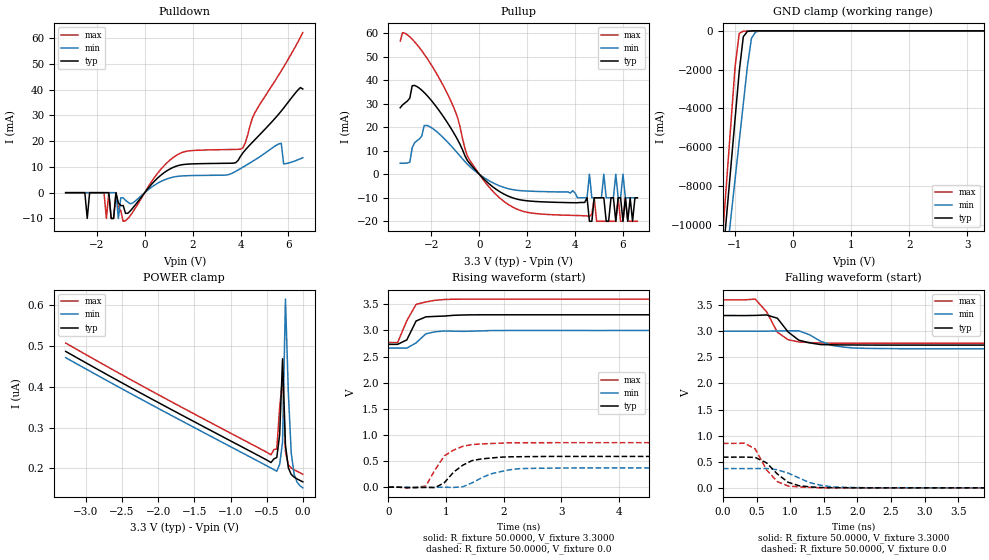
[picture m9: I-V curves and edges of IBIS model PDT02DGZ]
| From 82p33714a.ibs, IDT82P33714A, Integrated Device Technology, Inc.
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|   Model PDT02DGZ@
[Model]  PDT02DGZ
Model_type 3-state
Polarity   Non-Inverting
Enable   Active-Low
Vmeas =  1.6500V
Cref =   50.0000pF
Rref =   1.0000M
Vref =   0.0V
C_comp   70.4000fF   58.1000fF   75.7000fF
[Temperature Range]   25.0000   0.1250k   -40.0000
[Voltage Range]   3.3000V   3.0000V   3.6000V
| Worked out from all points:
|   slope of the pulldown table from 0 to 0.495 V, typ, clamps not added: 93.5 ohm
|   slope of the pullup table from 0 to 0.495 V, typ, clamps not added: 103 ohm
|   GND clamp passes 1 mA (typ) near -0.64 V on its own axis
|   rising waveform, R_fixture 50.0000, V_fixture 3.3000: 20-80 % time 160ps typ, 217ps min, 223ps max; typ from 2.73 V to 3.3 V
|   rising waveform, R_fixture 50.0000, V_fixture 0.0: 20-80 % time 384ps typ, 503ps min, 363ps max; typ from 0 V to 0.588 V
|   falling waveform, R_fixture 50.0000, V_fixture 3.3000: 20-80 % time 262ps typ, 328ps min, 254ps max; typ from 3.3 V to 2.73 V
|   falling waveform, R_fixture 50.0000, V_fixture 0.0: 20-80 % time 304ps typ, 438ps min, 266ps max; typ from 0.588 V to 0 V
[Pulldown]
|Voltage   I(typ)   I(min)   I(max)
-3.3V     0A         0A         0A
-2.5V     0A         0A         0A
-2.4V     -10mA      0A         0A
-1.6V     0A         0A         -10mA
-1.5V     0A         0A         0A
-1.4V     -10mA      0A         -10mA
-1.2V     0A         0A         0A
-1.1V     -4mA       -10mA      -6mA
-900mV    -5mA       -2mA       -11.11mA
1.3V      10.23mA    6.236mA    14.35mA
4.1V      15.46mA    9.888mA    17.41mA
6.6V      40.22mA    13.56mA    62.13mA
[Pullup]
|Voltage   I(typ)   I(min)   I(max)
-3.3V     28.25mA    4.655mA    56.59mA
-2.2V     33.66mA    20.75mA    49.56mA
-400mV    4.59mA     3.281mA    5.938mA
1V        -8.271mA   -5.504mA   -11.3mA
4.5V      -10mA      -10mA      -17.7mA
4.6V      -20mA      0A         -18mA
4.7V      -20mA      -10mA      -17mA
4.8V      -10mA      -10mA      -10mA
6V        -20mA      0A         -20mA
6.1V      -10mA      -10mA      -10mA
6.2V      -20mA      -10mA      -20mA
6.6V      -10mA      -10mA      -20mA
[GND_clamp]
|Voltage   I(typ)   I(min)   I(max)
-3.3V     -83.46A    -71.04A    -95.7A
-1.2V     -11.69A    -13.39A    -10.37A
-1.13V    -9.3A      -11.47A    -7.522A
-1.06V    -6.904A    -9.549A    -4.675A
-990mV    -4.509A    -7.624A    -1.828A
-920mV    -2.113A    -5.699A    -140.7mA
-850mV    -308.3mA   -3.775A    -17.61mA
-780mV    -30.18mA   -1.85A     -8.684mA
-710mV    -4.231mA   -388.3mA   -4.536mA
-640mV    -826.8uA   -62.95mA   -1.713mA
-430mV    -4.377uA   -246.1uA   -5.398uA
3.28V     165.3nA    264.6nA    156.9nA
[POWER_clamp]
|Voltage   I(typ)   I(min)   I(max)
-3.28V    486.2nA    470.9nA    506.6nA
-440mV    214.3nA    200.8nA    233.1nA
-400mV    223.3nA    196.9nA    246nA
-360mV    226.7nA    193nA      247.8nA
-320mV    282.8nA    210nA      349.4nA
-280mV    468.1nA    264.6nA    421.2nA
-240mV    257.3nA    614.1nA    241nA
-200mV    201.3nA    384.8nA    208.8nA
-160mV    185.2nA    237.6nA    200.8nA
-120mV    178.7nA    185.9nA    196.6nA
-80mV     174.4nA    166.5nA    192.9nA
0V        167.1nA    152.4nA    185.7nA
[Ramp]
| variable   typ   min   max
dV/dt_r  0.3530/0.3844n   0.2212/0.4930n   0.5110/0.3630n
dV/dt_f  0.3396/0.2623n   0.2022/0.3186n   0.4986/0.2510n
R_load = 50.0000
[Rising Waveform]
R_fixture= 50.0000
V_fixture= 3.3000
V_fixture_min= 3.0000
V_fixture_max= 3.6000
L_fixture= 0.0H
C_fixture= 0.0F
|time   V(typ)   V(min)   V(max)
0s        2.734V     2.663V     2.769V
160ps     2.734V     2.663V     2.768V
320ps     2.82V      2.662V     3.188V
480ps     3.181V     2.762V     3.499V
650ps     3.261V     2.936V     3.546V
810ps     3.269V     2.975V     3.578V
970ps     3.276V     2.99V      3.593V
1.29ns    3.296V     2.983V     3.599V
1.62ns    3.3V       2.992V     3.599V
16ns      3.3V       3V         3.6V
[Rising Waveform]
R_fixture= 50.0000
V_fixture= 0.0
V_fixture_min= 0.0
V_fixture_max= 0.0
L_fixture= 0.0H
C_fixture= 0.0F
|time   V(typ)   V(min)   V(max)
0s        7.011uV    7.347uV    6.889uV
650ps     -2.872mV   -5.444mV   22.73mV
810ps     -8.827mV   -2.518mV   335.1mV
970ps     85.14mV    -1.489mV   599.3mV
1.13ns    288.1mV    -5.225mV   709.9mV
1.29ns    421.3mV    8.1mV      782.5mV
1.62ns    541.9mV    182.4mV    828.5mV
2.1ns     581mV      332.4mV    850.5mV
2.59ns    586.5mV    361.9mV    851.3mV
16ns      588.4mV    368.7mV    851.6mV
[Falling Waveform]
R_fixture= 50.0000
V_fixture= 3.3000
V_fixture_min= 3.0000
V_fixture_max= 3.6000
L_fixture= 0.0H
C_fixture= 0.0F
|time   V(typ)   V(min)   V(max)
0s        3.3V       3V         3.6V
480ps     3.302V     2.999V     3.614V
650ps     3.311V     3V         3.372V
810ps     3.248V     3.004V     2.98V
970ps     2.985V     3.007V     2.837V
1.13ns    2.827V     3.007V     2.794V
1.45ns    2.744V     2.809V     2.773V
1.78ns    2.737V     2.698V     2.77V
2.59ns    2.734V     2.665V     2.769V
16ns      2.734V     2.663V     2.769V
[Falling Waveform]
R_fixture= 50.0000
V_fixture= 0.0
V_fixture_min= 0.0
V_fixture_max= 0.0
L_fixture= 0.0H
C_fixture= 0.0F
|time   V(typ)   V(min)   V(max)
0s        588.4mV    368.7mV    851.7mV
320ps     588.8mV    368.6mV    854.8mV
480ps     582.9mV    368.8mV    746.5mV
650ps     478.5mV    371.4mV    342.9mV
810ps     265mV      346.2mV    119.4mV
970ps     107.2mV    282.7mV    35.4mV
1.29ns    19.2mV     99.89mV    8.654mV
1.62ns    3.531mV    18.39mV    397.3uV
2.26ns    -68.31uV   501uV      90.27uV
16ns      -5.204uV   -6.912uV   12.02uV
